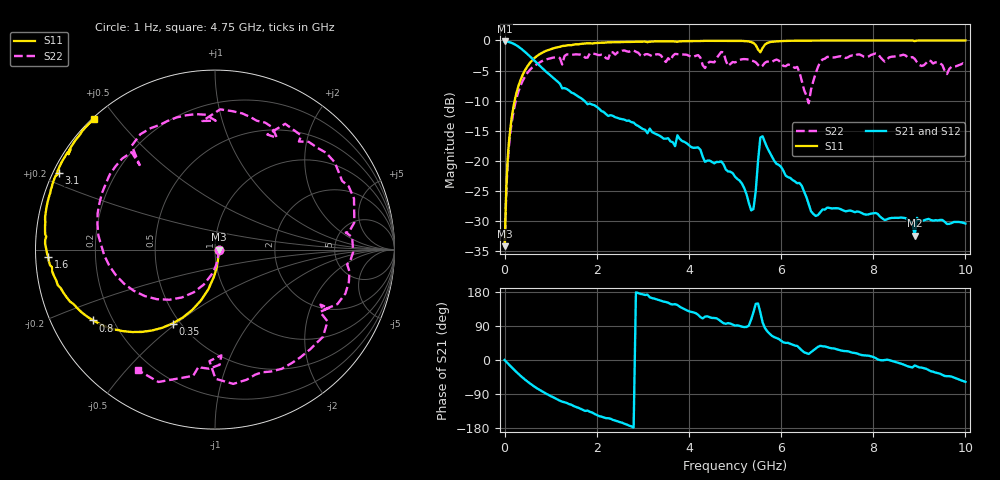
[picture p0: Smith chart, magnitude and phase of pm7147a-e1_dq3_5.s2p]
# GHz S DB R 50
! S-Parameters data
! Freq  dbS11  angS11  dbS21  angS21  dbS12  angS12  dbS22  angS22
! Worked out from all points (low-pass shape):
!   279 points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, 1 Hz to 10 GHz, reference 50 ohm
!   highest |S21| = -0.17 dB at 7.943 kHz (marker M1); lowest = -32.4 dB at 8.9 GHz (marker M2)
!   |S21| within 3 dB of the highest: start of sweep to 621.1 MHz
!   lowest |S11| = -34.1 dB at 3.981 kHz (marker M3), VSWR 1.04, Z = 52 - j0.000613 ohm
!   |S11| at or under -10 dB: start of sweep to 219 MHz
!   |S22| runs from -34.1 to -1.7 dB; largest |S21 - S12| = 0
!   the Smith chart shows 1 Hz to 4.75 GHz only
!   S11 on the Smith chart (normalised r, x): 1 Hz: 1.04, -0.00; 350 MHz: 0.46, -0.48; 800 MHz: 0.13, -0.27; 1.6 GHz: 0.04, -0.02; 3.1 GHz: 0.02, +0.23; 4.75 GHz: 0.00, +0.44
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1e-09  -34.13 -0.0  -0.17 -0.0  -0.17 -0.0  -34.13 -0.0
3.9811e-06  -34.13 -0.0  -0.17 -0.0  -0.17 -0.0  -34.13 -0.0
7.9433e-06  -34.13 -0.0  -0.17 -0.0  -0.17 -0.0  -34.13 -0.0
0.1  -16.37 -92.3  -0.28 -12.7  -0.28 -12.7  -17.15 -97.4
0.35  -6.47 -119.9  -1.32 -42.1  -1.32 -42.1  -7.42 -139.5
0.8  -2.11 -149.8  -4.48 -81.9  -4.48 -81.9  -3.48 167.8
1.6  -0.64 -177.3  -9.32 -126.0  -9.32 -126.0  -2.33 102.1
1.7  -0.55 -179.7  -9.82 -131.6  -9.82 -131.6  -2.46 93.9
2.3  -0.31 167.9  -12.40 -155.0  -12.40 -155.0  -1.91 60.8
3.1  -0.29 153.8  -15.40 172.5  -15.40 172.5  -2.27 -1.1
3.35  -0.15 151.3  -15.76 158.0  -15.76 158.0  -2.31 -18.6
4.2  -0.11 140.0  -17.75 119.3  -17.75 119.3  -2.44 -82.2
4.75  -0.07 132.9  -20.54 97.2  -20.54 97.2  -1.97 -122.6
5.05  -0.07 128.8  -22.98 91.4  -22.98 91.4  -3.49 -134.1
5.4  -0.42 121.4  -27.98 125.8  -27.98 125.8  -3.43 -162.8
5.6  -1.25 130.5  -15.91 98.9  -15.91 98.9  -4.18 -168.4
6.4  -0.05 118.1  -23.65 31.4  -23.65 31.4  -5.31 132.1
6.7  -0.03 115.1  -28.79 25.3  -28.79 25.3  -6.74 161.7
7.3  -0.01 109.5  -28.02 25.0  -28.02 25.0  -2.61 118.1
8.35  -0.01 101.0  -29.51 -0.4  -29.51 -0.4  -2.79 72.3
8.9  -0.12 96.1  -32.37 -14.3  -32.37 -14.3  -3.06 37.2
10  -0.01 89.9  -30.38 -57.7  -30.38 -57.7  -3.95 -26.7
